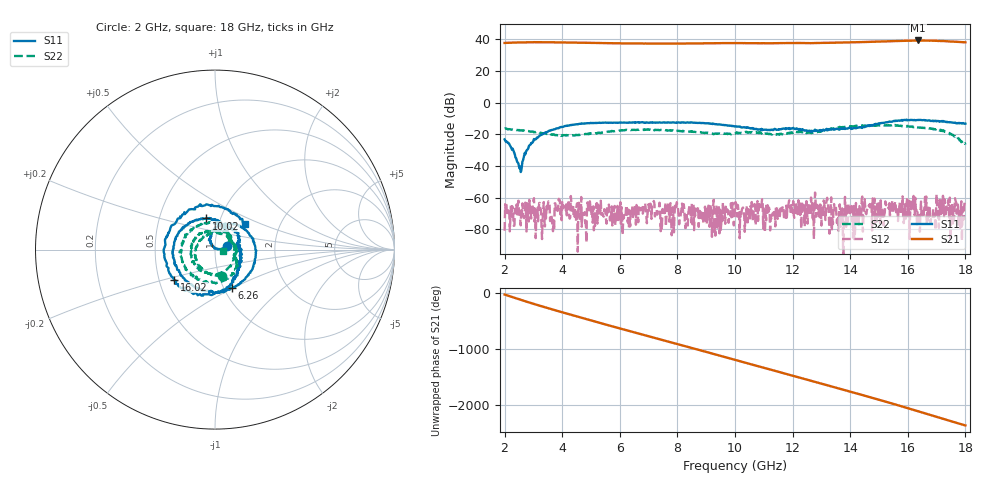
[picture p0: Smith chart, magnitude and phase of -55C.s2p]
!Agilent Technologies,E8361C,US49010292,A.09.42.06
!Agilent E8361C: A.09.42.06
!Date: Wednesday, June 03, 2026 23:02:01
!Correction: S11(Full 2 Port(1,2))
!S21(Full 2 Port(1,2))
!S12(Full 2 Port(1,2))
!S22(Full 2 Port(1,2))
!S2P File: Measurements: S11, S21, S12, S22:
# Hz S  dB  R 50
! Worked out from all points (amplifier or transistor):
!   801 points, 2 GHz to 18 GHz, reference 50 ohm
!   highest |S21| = 39.3 dB at 16.36 GHz (marker M1)
!   |S21| within 3 dB of that: start of sweep to end of sweep
!   unconditionally stable (mu >= 1): start of sweep to end of sweep
!   at 4.66 GHz: K = 5.76, MAG = 38.2 dB, |S12| = -59.6 dB
!   at 10 GHz: K = 15.54, MAG = 37.9 dB, |S12| = -67.9 dB
!   at 18 GHz: K = 6.69, MAG = 38.4 dB, |S12| = -61.1 dB
!   S11 on the Smith chart (normalised r, x): 2 GHz: 1.14, +0.04; 6.26 GHz: 1.09, -0.49; 10.02 GHz: 0.86, +0.31; 16.02 GHz: 0.60, -0.22; 18 GHz: 1.34, +0.39
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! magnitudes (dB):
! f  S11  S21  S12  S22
! 2 GHz  -23.2  37.8  -80.9  -16.3
! 2.54 GHz  -40.3  38.1  -73.2  -17.5
! 3.2 GHz  -21.2  38.2  -63.4  -18.6
! 4.68 GHz  -13.2  37.9  -78.4  -20.0
! 6.26 GHz  -12.6  37.5  -73.3  -17.3
! 7.34 GHz  -12.5  37.4  -66.5  -17.2
! 10 GHz  -15.1  37.7  -67.9  -19.5
! 10.02 GHz  -14.9  37.7  -62.7  -19.1
! 12.68 GHz  -18.2  37.7  -63.6  -19.0
! 13.68 GHz  -16.3  38.0  -68.4  -15.8
! 13.96 GHz  -15.8  38.1  -64.0  -14.9
! 14.14 GHz  -16.0  38.2  -86.2  -14.8
! 14.66 GHz  -14.8  38.4  -64.5  -14.4
! 15.34 GHz  -12.1  38.8  -66.9  -14.3
! 16.02 GHz  -11.0  39.2  -71.9  -14.9
! 16.18 GHz  -11.0  39.3  -62.6  -15.1
! 16.36 GHz  -10.9  39.3  -68.7  -15.7
! 16.56 GHz  -10.9  39.3  -68.4  -15.8
! 16.88 GHz  -11.7  39.2  -67.2  -16.8
! 17.22 GHz  -11.5  39.0  -58.8  -17.7
! 17.84 GHz  -12.9  38.3  -67.7  -24.2
! 18 GHz  -13.2  38.2  -61.1  -26.5
